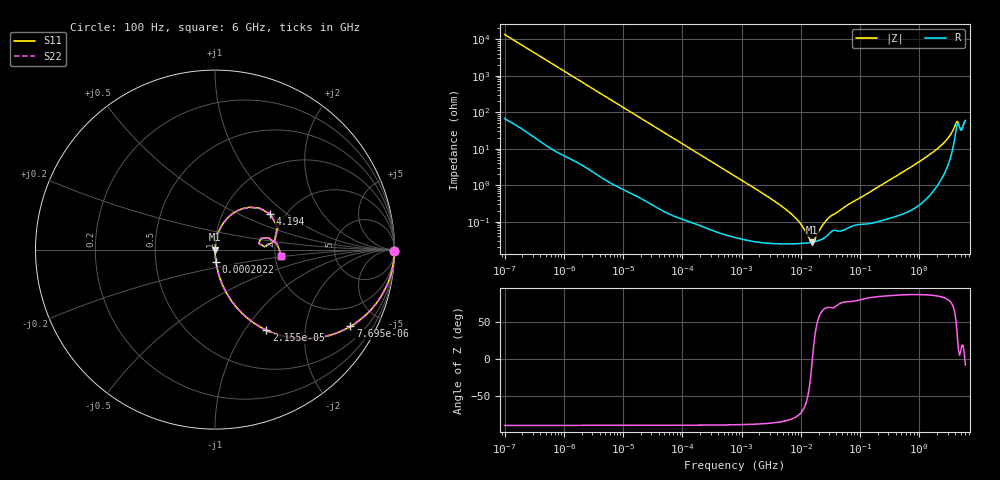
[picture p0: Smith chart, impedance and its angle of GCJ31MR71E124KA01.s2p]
!Murata Part Number: GCJ31MR71E124KA01
!These Parameters are Measured in Series Mode Connection
!Data Generated on Mar 13, 2026
!  o--ll--o
!Port1  Port2
!  o------o
!Operation Temp=25[degC], DC Bias Voltage=0[V]
!Freq. Start=100[Hz] Stop=6[GHz] 401[Steps]
# Hz S RI R 50
!Freq.(Hz) S11(Real) S11(Imag) S21(Real) S21(Imag) S12(Real) S12(Imag) S22(Real) S22(Imag)
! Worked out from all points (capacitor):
!   401 points, 100 Hz to 6 GHz, reference 50 ohm
!   read as one part in series: C = 119 nF near 109 Hz
!   lowest |Z| = 27.7 mohm at 15.56 MHz (marker M1)
!   series resonance near 15.7 MHz, so ESL is about 860 pH
!   S11 on the Smith chart (normalised r, x): 100 Hz: open; 7.695 kHz: 1.02, -3.52; 21.55 kHz: 1.01, -1.26; 202.2 kHz: 1.00, -0.14; 4.194 GHz: 1.67, +0.77; 6 GHz: 2.17, -0.17
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100  0.9999 -0.00748  9.34e-05 0.00748  9.34e-05 0.00748  0.9999 -0.00748
2008  0.9776 -0.1455  0.0224 0.1455  0.0224 0.1455  0.9776 -0.1455
4299  0.907 -0.2879  0.093 0.2879  0.093 0.2879  0.907 -0.2879
7695  0.7548 -0.4275  0.2452 0.4275  0.2452 0.4275  0.7548 -0.4275
13169  0.5148 -0.4968  0.4852 0.4968  0.4852 0.4968  0.5148 -0.4968
21550  0.286 -0.4487  0.714 0.4487  0.714 0.4487  0.286 -0.4487
40335  0.1041 -0.302  0.8959 0.302  0.8959 0.302  0.1041 -0.302
202169  0.00535 -0.0674  0.9947 0.0674  0.9947 0.0674  0.00535 -0.0674
774597  0.000687 -0.0178  0.9993 0.0178  0.9993 0.0178  0.000687 -0.0178
6353432  0.000251 -0.00183  0.9997 0.00183  0.9997 0.00183  0.000251 -0.00183
9506416  0.000254 -0.000929  0.9997 0.000929  0.9997 0.000929  0.000254 -0.000929
1.555665e7  0.000276 -1.58e-05  0.9997 1.58e-05  0.9997 1.58e-05  0.000276 -1.58e-05
1.701401e7  0.000285 0.000144  0.9997 -0.000144  0.9997 -0.000144  0.000285 0.000144
2.434276e7  0.000356 0.000814  0.9996 -0.000814  0.9996 -0.000814  0.000356 0.000814
3.184506e7  0.000519 0.00133  0.9995 -0.00133  0.9995 -0.00133  0.000519 0.00133
3.124326e8  0.00142 0.0136  0.9986 -0.0136  0.9986 -0.0136  0.00142 0.0136
1.251881e9  0.00701 0.0556  0.993 -0.0556  0.993 -0.0556  0.00701 0.0556
2.562649e9  0.0366 0.1325  0.9634 -0.1325  0.9634 -0.1325  0.0366 0.1325
3.352442e9  0.0972 0.1998  0.9028 -0.1998  0.9028 -0.1998  0.0972 0.1998
4.193612e9  0.3075 0.1989  0.6925 -0.1989  0.6925 -0.1989  0.3075 0.1989
5.016141e9  0.2443 0.0352  0.7557 -0.0352  0.7557 -0.0352  0.2443 0.0352
6e9  0.3703 -0.0346  0.6297 0.0346  0.6297 0.0346  0.3703 -0.0346
